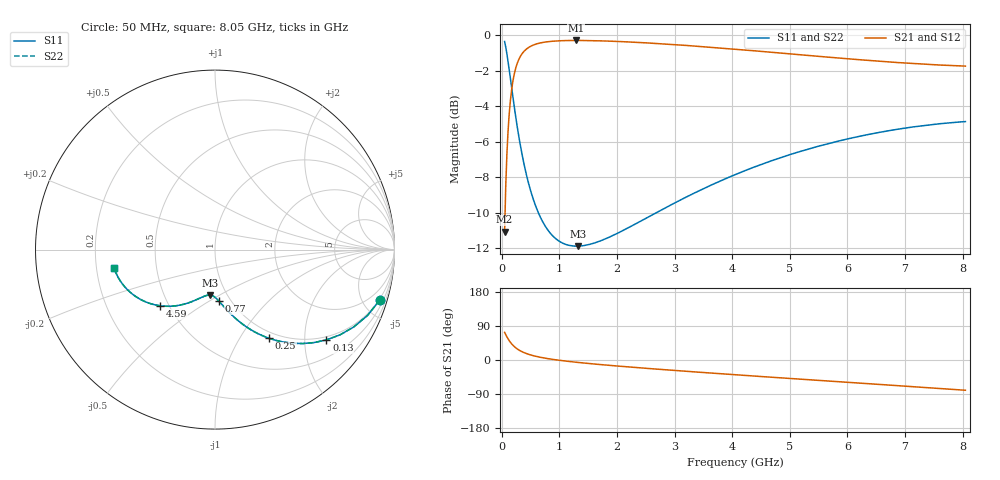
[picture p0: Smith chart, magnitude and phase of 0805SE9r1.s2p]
! AVX Thin Film Operation		Date: August 2001
! Description: Accu-P® Series, Thin Film, SMD, RF Capacitor
! Part Number: 08051J9R1BBT
! 50 MHz  -  8.05 GHz
! Serial Measurements
# mhz S db R 50
!	S11		S21		S12		S22
!	dB	Phase	dB	Phase	dB	Phase	dB	Phase
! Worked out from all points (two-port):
!   401 points, 50 MHz to 8.05 GHz, reference 50 ohm
!   highest |S21| = -0.29 dB at 1.29 GHz (marker M1); lowest = -11.1 dB at 50 MHz (marker M2)
!   |S21| within 3 dB of the highest: 163.8 MHz to end of sweep
!   lowest |S11| = -11.9 dB at 1.33 GHz (marker M3), VSWR 1.68, Z = 41.7 - j22.6 ohm
!   |S11| at or under -10 dB: 637.1 MHz to 2.679 GHz (2.041 GHz wide, 123 % of centre)
!   |S22| runs from -11.9 to -0.4 dB; largest |S21 - S12| = 0
!   S11 on the Smith chart (normalised r, x): 50 MHz: 0.91, -6.54; 130 MHz: 0.91, -2.54; 250 MHz: 0.91, -1.35; 770 MHz: 0.88, -0.55; 4.59 GHz: 0.45, -0.35; 8.05 GHz: 0.27, -0.08
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50  -0.35 -17.1  -11.05 72.9  -11.05 72.9  -0.35 -17.1
90  -1.05 -29.1  -6.68 60.9  -6.68 60.9  -1.05 -29.1
110  -1.49 -34.3  -5.39 55.7  -5.39 55.7  -1.49 -34.3
130  -1.95 -39.0  -4.42 51.0  -4.42 51.0  -1.95 -39.0
150  -2.43 -43.3  -3.69 46.7  -3.69 46.7  -2.43 -43.3
190  -3.39 -50.4  -2.67 39.6  -2.67 39.6  -3.39 -50.4
250  -4.75 -58.6  -1.77 31.3  -1.77 31.3  -4.75 -58.6
330  -6.32 -66.4  -1.16 23.6  -1.16 23.6  -6.32 -66.4
430  -7.87 -73.0  -0.78 16.9  -0.78 16.9  -7.87 -73.1
590  -9.62 -80.1  -0.50 9.8  -0.50 9.8  -9.62 -80.2
770  -10.82 -85.6  -0.38 4.4  -0.38 4.4  -10.82 -85.6
1010  -11.62 -90.9  -0.31 -1.0  -0.31 -1.0  -11.62 -90.9
1290  -11.87 -95.8  -0.29 -5.9  -0.29 -5.9  -11.87 -95.8
1330  -11.88 -96.4  -0.29 -6.5  -0.29 -6.5  -11.88 -96.5
1390  -11.86 -97.4  -0.30 -7.5  -0.30 -7.5  -11.86 -97.4
1990  -11.18 -105.6  -0.35 -15.7  -0.35 -15.7  -11.18 -105.6
2730  -9.91 -114.4  -0.47 -24.5  -0.47 -24.5  -9.91 -114.4
4050  -7.85 -128.8  -0.79 -38.9  -0.79 -38.9  -7.85 -128.8
4590  -7.17 -134.4  -0.93 -44.5  -0.93 -44.5  -7.17 -134.4
5390  -6.35 -142.6  -1.16 -52.7  -1.16 -52.7  -6.35 -142.6
6730  -5.37 -156.1  -1.51 -66.2  -1.51 -66.2  -5.37 -156.1
8050  -4.86 -169.6  -1.74 -79.8  -1.74 -79.8  -4.86 -169.7
